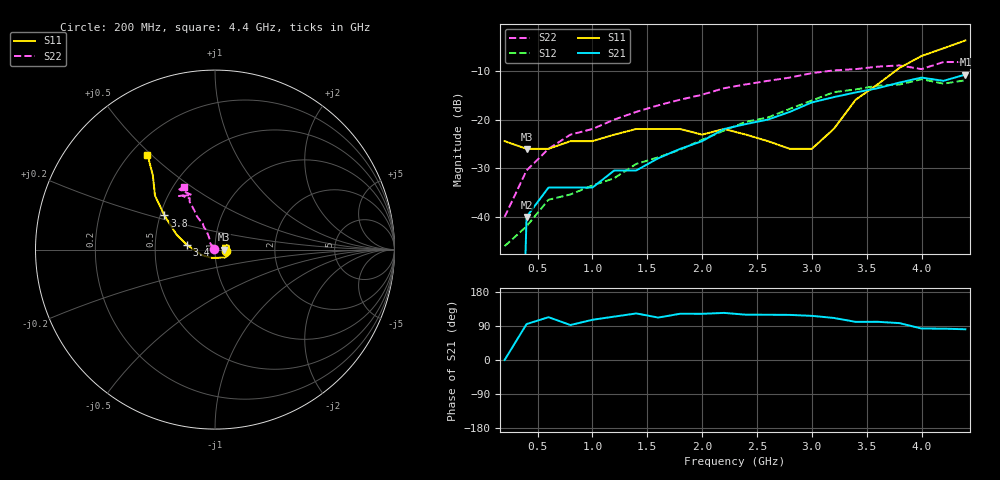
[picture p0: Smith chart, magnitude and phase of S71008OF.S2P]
!  MGS-71008 S PARAMETERS
!  "off" port  LAST UPDATED 07-22-92
# ghz s ma r 50
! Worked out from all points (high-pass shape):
!   22 points, 200 MHz to 4.4 GHz, reference 50 ohm
!   highest |S21| = -10.75 dB at 4.4 GHz (marker M1); lowest = -40.0 dB at 400 MHz (marker M2)
!   |S21| within 3 dB of the highest: 3.555 GHz to end of sweep
!   lowest |S11| = -26.0 dB at 400 MHz (marker M3), VSWR 1.11, Z = 55.3 + j0 ohm
!   |S11| at or under -10 dB: start of sweep to 3.763 GHz
!   |S22| runs from -40.0 to -8.2 dB; largest |S21 - S12| = 0.048
!   S11 on the Smith chart (normalised r, x): 200 MHz: 1.13, -0.02; 3.4 GHz: 0.73, +0.04; 3.8 GHz: 0.53, +0.23; 4.4 GHz: 0.27, +0.49
0.2  0.06 -9.8  0 73.6  0.005 74.7  0.01 146.5
0.4  0.05 0.0  0.01 94.8  0.008 95.5  0.03 130.7
0.6  0.05 27.3  0.02 113.0  0.015 113.7  0.05 125.1
0.8  0.06 20.7  0.02 92.3  0.017 93.0  0.07 116.9
1  0.06 21.7  0.02 106.1  0.021 107.1  0.08 115.7
1.2  0.07 20.6  0.03 114.5  0.025 116.4  0.1 114.8
1.4  0.08 15.7  0.03 122.9  0.035 125.5  0.12 114.6
1.6  0.08 -5.6  0.04 112.0  0.041 114.2  0.14 116.3
1.8  0.08 -11.8  0.05 122.0  0.049 124.9  0.16 115.2
2  0.07 -17.0  0.06 121.9  0.062 125.4  0.18 117.1
2.2  0.08 -24.6  0.08 124.3  0.077 128.3  0.21 118.5
2.4  0.07 -40.0  0.09 119.5  0.095 123.5  0.23 117.9
2.6  0.06 -46.7  0.1 119.4  0.105 124.0  0.25 117.8
2.8  0.05 -66.2  0.12 119.0  0.129 122.9  0.27 117.9
3  0.05 -112.4  0.15 116.5  0.157 119.7  0.3 118.0
3.2  0.08 -158.0  0.17 111.0  0.191 113.1  0.32 116.2
3.4  0.16 170.2  0.19 100.7  0.204 100.3  0.33 119.8
3.6  0.23 158.7  0.21 100.8  0.223 96.7  0.35 120.5
3.8  0.34 146.0  0.24 97.3  0.229 90.9  0.36 124.0
4  0.45 138.0  0.27 83.0  0.26 78.3  0.33 113.0
4.2  0.54 129.9  0.25 82.7  0.234 78.8  0.39 120.7
4.4  0.65 125.4  0.29 81.1  0.253 74.5  0.39 116.1
